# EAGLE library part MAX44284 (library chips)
A precision current amplifier that can do low or high side sensing
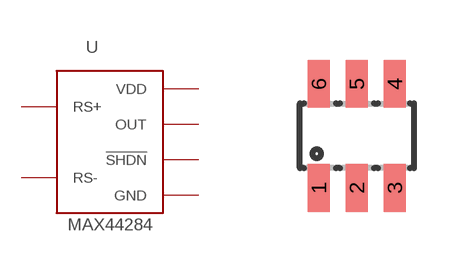
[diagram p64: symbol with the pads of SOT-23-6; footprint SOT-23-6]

Designator prefix -

## MAX44284 (DIGIKEY: MAX44284FAUT+TCT-ND)  [SOT-23-6]
1  VDD
2  GND
3  RS+
4  RS-
5  OUT
6  !SHDN

## Footprint SOT-23-6 (pad centres in mm)
Small Outline Transistor
smd 0.55 x 1.2: 1 -0.95,-1.3; 2 0,-1.3; 3 0.95,-1.3; 4 0.95,1.3; 5 0,1.3; 6 -0.95,1.3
